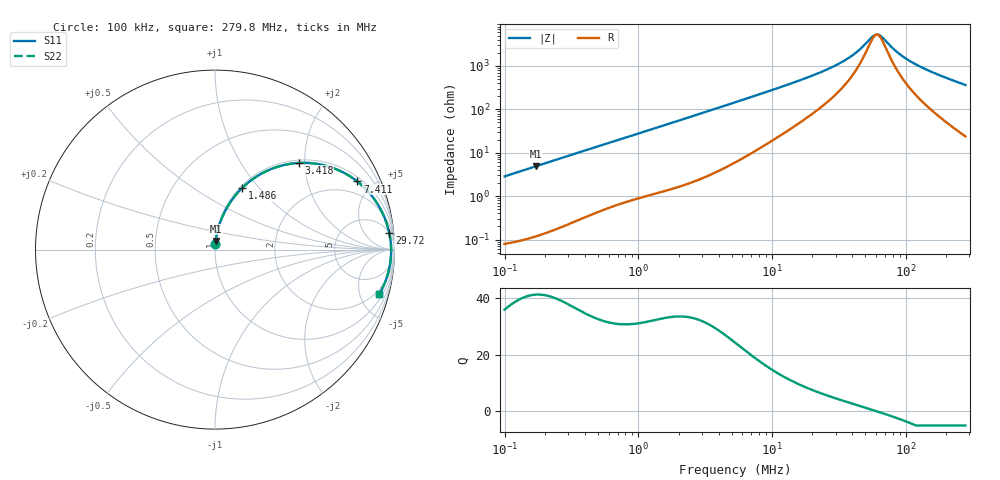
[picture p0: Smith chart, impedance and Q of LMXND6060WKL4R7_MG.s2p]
! LMXND6060WKL4R7_MG  S-PARAMETER MODEL  ( General Type )
! Model Generated by TAIYO YUDEN Corporation (https://www.yuden.co.jp/en/)
! Version 1.0
! TAIYO YUDEN Control No. 191025NI43SB-FBB
! Copyright(c) 2019 TAIYO YUDEN CO.,LTD. All Rights Reserved.
! Product Description (link to TY-COMPAS)
! https://ds.yuden.co.jp/TYCOMPAS/or/detail?pn=LMXND6060WKL4R7NMG&u=M
! Products Name : Inductors
! Characteristics :
!  Inductance : 4.7 uH , SRF(min) : 43 MHz , DC Resistance(max) : 0.0696 Ohm
!  Rated Current : Saturation :2400 mA , Temp Rise : 2150 mA (40 degC)
!  Case Size : 6.0 x 6.0 / 0.236 x 0.236 [mm/inch] , Thickness : 2 / 0.079 [mm/inch]
!  (Conditions: Temperature = 25 degC , DC Bias Current/Voltage = 0A / 0V)
! External Node Assignments :
!  1  o---GGG---o  2
! GND o---------o GND
! Frequency Range : 0.1MHz  -  279.750408MHz  [ 402 STEP ]
# MHz S RI R 50
! Freq[MHz].  S11 Real  S11 Imag  S21 Real  S21 Imag  S12 Real  S12 Imag  S22 Real  S22 Imag
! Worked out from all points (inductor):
!   401 points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, 100 kHz to 279.8 MHz, reference 50 ohm
!   read as one part in series: L = 4.53 uH near 104 kHz
!   highest Q = 41.3 at 170.9 kHz (marker M1), where L = 4.53 uH
!   self-resonance near 60.87 MHz
!   S11 on the Smith chart (normalised r, x): 100 kHz: 1.00, +0.06; 1.486 MHz: 1.02, +0.81; 3.418 MHz: 1.06, +1.86; 7.411 MHz: 1.21, +4.07; 29.72 MHz: 5, +20; 279.8 MHz: 1.47, -7.25
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0.1  0.0016 0.0284  0.9984 -0.0284  0.9984 -0.0284  0.0016 0.0284
0.170867  0.00353 0.0484  0.9965 -0.0484  0.9965 -0.0484  0.00353 0.0484
0.377863  0.0142 0.1048  0.9858 -0.1048  0.9858 -0.1048  0.0142 0.1048
0.819208  0.0554 0.213  0.9446 -0.213  0.9446 -0.213  0.0554 0.213
1.427803  0.1405 0.3325  0.8595 -0.3325  0.8595 -0.3325  0.1405 0.3325
1.485601  0.1497 0.3419  0.8503 -0.3419  0.8503 -0.3419  0.1497 0.3419
2.209228  0.2727 0.4307  0.7273 -0.4307  0.7273 -0.4307  0.2727 0.4307
3.418322  0.4659 0.4828  0.5341 -0.4828  0.5341 -0.4828  0.4659 0.4828
5.289144  0.6697 0.4502  0.3303 -0.4502  0.3303 -0.4502  0.6697 0.4502
7.410937  0.7933 0.3794  0.2067 -0.3794  0.2067 -0.3794  0.7933 0.3794
11.69668  0.8971 0.2672  0.1029 -0.2672  0.1029 -0.2672  0.8971 0.2672
19.9857  0.9531 0.1553  0.0469 -0.1553  0.0469 -0.1553  0.9531 0.1553
29.72063  0.9711 0.0916  0.0289 -0.0916  0.0289 -0.0916  0.9711 0.0916
40.82525  0.9782 0.0488  0.0218 -0.0488  0.0218 -0.0488  0.9782 0.0488
56.07892  0.9812 0.00985  0.0188 -0.00985  0.0188 -0.00985  0.9812 0.00985
59.51829  0.9814 0.0027  0.0186 -0.0027  0.0186 -0.0027  0.9814 0.0027
64.43445  0.9815 -0.00684  0.0185 0.00684  0.0185 0.00684  0.9815 -0.00684
75.51853  0.9811 -0.0261  0.0189 0.0261  0.0189 0.0261  0.9811 -0.0261
93.93766  0.979 -0.0538  0.021 0.0538  0.021 0.0538  0.979 -0.0538
121.5793  0.9739 -0.0896  0.0261 0.0896  0.0261 0.0896  0.9739 -0.0896
177.248  0.9583 -0.1515  0.0417 0.1515  0.0417 0.1515  0.9583 -0.1515
279.7504  0.9158 -0.247  0.0842 0.247  0.0842 0.247  0.9158 -0.247
